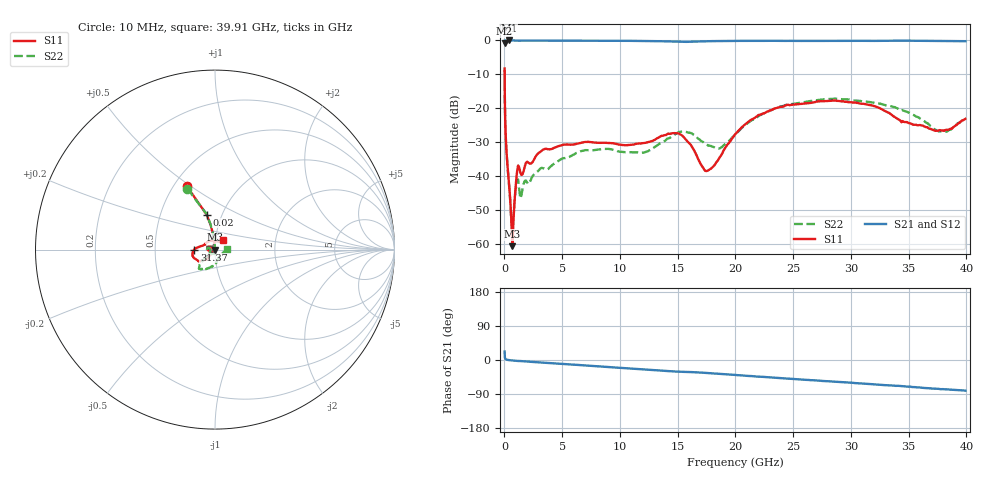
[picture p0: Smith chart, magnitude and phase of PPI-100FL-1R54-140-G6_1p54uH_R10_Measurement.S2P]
! Data measured by Modelithics Inc.  support@modelithics.com  813-866-6335  Tampa FL USA June 2025
! PPI-100FL-1R54-140-G6_1p54uH measured on 10-mil thick RO4350B board, mounted in 2-port shunt configuration on a 50-ohm transmission line
# Hz S MA R 50
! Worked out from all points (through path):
!   429 points, 10 MHz to 39.91 GHz, reference 50 ohm
!   highest |S21| = -0.01 dB at 397.1 MHz (marker M1); lowest = -0.8 dB at 10 MHz (marker M2)
!   group delay of S21, straight-line fit = 5.65 ps
!   lowest |S11| = -60.5 dB at 688.4 MHz (marker M3), VSWR 1.00, Z = 49.9 - j0.0213 ohm
!   |S11| at or under -10 dB: 13.07 MHz to end of sweep
!   |S22| runs from -56.5 to -8.6 dB; largest |S21 - S12| = 0.025
!   S11 on the Smith chart (normalised r, x): 10 MHz: 0.58, +0.48; 20 MHz: 0.85, +0.34; 31.37 GHz: 0.79, +0.00; 39.91 GHz: 1.08, +0.12
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1e7  0.3866 114.0  0.9129 22.2  0.913 22.2  0.3717 114.4
2e7  0.2007 103.4  0.9742 11.6  0.9742 11.6  0.202 103.2
7e7  0.05935 96.3  0.996 3.3  0.996 3.3  0.05927 95.5
2e8  0.01983 96.5  0.9985 0.8  0.9986 0.8  0.01971 94.3
3.970888e8  0.007616 101.4  0.9989 -0.3  0.999 -0.3  0.007378 98.1
4.941776e8  0.004618 106.4  0.9989 -0.6  0.999 -0.7  0.004418 104.2
6.883552e8  0.0009408 -166.9  0.9988 -1.3  0.9989 -1.3  0.001496 -171.9
1.07671e9  0.01132 -103.4  0.9947 -2.5  0.995 -2.5  0.008621 -136.8
1.270888e9  0.01364 -137.0  0.9908 -2.6  0.991 -2.6  0.006499 -165.4
3.406841e9  0.02503 -127.6  0.99 -7.1  0.9904 -7.1  0.01313 -108.0
6.70786e9  0.03137 -136.5  0.9893 -13.8  0.9894 -13.8  0.02371 -88.8
1.340699e10  0.03792 -173.3  0.9747 -27.9  0.9748 -28.0  0.03013 -126.2
1.534876e10  0.04029 157.8  0.9535 -31.0  0.9536 -31.1  0.04548 -169.3
1.748472e10  0.01195 175.8  0.9728 -34.1  0.973 -34.1  0.02964 168.7
1.864978e10  0.0192 -141.7  0.9808 -36.7  0.9809 -36.5  0.02584 -165.0
2.000902e10  0.04234 -131.4  0.9848 -39.5  0.985 -39.6  0.04191 -142.0
2.292169e10  0.09235 -138.3  0.9876 -45.7  0.9877 -45.7  0.09166 -137.8
2.670815e10  0.1222 -155.4  0.9831 -53.3  0.9832 -53.3  0.1301 -132.9
3.136841e10  0.1147 179.8  0.9853 -63.0  0.9855 -63.0  0.1256 -118.7
3.331019e10  0.08571 168.4  0.9877 -66.8  0.9879 -67.0  0.1077 -108.6
3.777627e10  0.04762 84.9  0.9788 -77.0  0.9791 -76.0  0.04576 -48.4
3.991223e10  0.0702 51.9  0.9742 -80.9  0.9744 -80.4  0.06943 1.3
